| TEXAS INSTRUMENTS INCORPORATED
| Standard Linear and Logic Group
| IBIS Model of SN74CBT16292
| 12-BIT 1-OF-2 FET MULTIPLEXER/DEMULTIPLEXER WITH INTERNAL PULLDOWN RESISTORS
| This file contains package information for the following:
|  TSSOP 56-pin (DGG) package as [Component] CBT16292_DGG
|  TVSOP 56-pin (DGV) package as [Component] CBT16292_DGV
|  SSOP 56-pin (DL) package as [Component] CBT16292_DL
| This device can be powered at the following Vccs:
|  4 volt Vcc
|  5 volt Vcc
| This file provides unique models under the [Model Selector] for each Vcc.
| For operation at a specific Vcc, select the appropriate model after each
| [Model Selector] keyword.
[IBIS Ver]   3.2
[Comment char]  |_char
[File Name]   sn74cbt16292.ibs
[File Rev]   1.1 | b_die
[Date]   January 16, 2004
[Source]   Data created from TI-SPICE simulations at TI-SLL.
[Notes]   The following is an IBIS list for the CBT16292.
   Please contact sllibis@ti.com with questions and
   comments concerning SLL IBIS models.
   - Power-clamp data has been deleted from the input model
   since there is no power-clamp diode.
   - Power Clamp never becomes zero due to internal pulldown
   resistors.
   - Non-monotonic data due to FET characteristics.
[Disclaimer] Property of Texas Instruments Incorporated.  Unauthorized
   reproduction and/or distribution is strictly prohibited.
   This product is protected under copyright law.
   Created  2002, (C) Copyright  2002, Texas Instruments
   Incorporated, All Rights Reserved
   UNLESS THERE IS A SIGNED, WRITTEN AGREEMENT TO THE
   CONTRARY, TEXAS INSTRUMENTS (TI) IS PROVIDING THE IBIS
   MODELS  AND WITHOUT ANY WARRANTY, EXPRESSED OR
   IMPLIED.  TI assumes no liability for:
   1) the accuracy of the IBIS models provided to your
   company;
   2) the proper functioning of these IBIS Models in your
   design or for any resulting applications; or
   3) infringement of patents, copyrights or intellectual
   property rights resulting from your use of these IBIS
   models.
   TI provides IBIS Models as a service to our customers.
   You and your company shall not distribute, sell or give
   these models to anyone else without prior written
   permission from TI.
   TI reserves the right to make changes to our products or
   to discontinue any semiconductor product or service
   without notice, and advises our customers to obtain the
   latest version of relevant information to verify, before
   placing orders, that the information being relied on is
   current.
   Please be aware that your receipt and use of the IBIS
   information provided shall serve as acceptance of these
   terms and conditions.  If you do not accept these terms,
   you should return or destroy the IBIS models and any
   other accompanying information immediately.
| Component CBT16292_DGG 56-pin TSSOP
[Component]   CBT16292_DGG
[Manufacturer]   Texas Instruments, Inc.
[Package]
|   typ   min   max
R_pkg   4.500e-02   3.500e-02   6.200e-02
L_pkg   3.324e-09   2.403e-09   5.094e-09
C_pkg   5.640e-13   3.410e-13   9.140e-13
[Pin]   signal_name   model_name   R_pin   L_pin   C_pin
1   S   CBT16292_IN   6.200e-02   5.094e-09   8.560e-13
2   1A   CBT16292_IO   6.100e-02   4.621e-09   9.020e-13
3   NC   NC   6.000e-02   4.316e-09   8.020e-13
4   2A   CBT16292_IO   5.900e-02   3.968e-09   6.980e-13
5   NC   NC   5.700e-02   3.716e-09   6.490e-13
6   3A   CBT16292_IO   4.200e-02   3.517e-09   6.520e-13
7   NC   NC   4.100e-02   3.160e-09   5.700e-13
8   GND   GND   3.900e-02   2.981e-09   4.820e-13
9   4A   CBT16292_IO   3.900e-02   2.809e-09   4.470e-13
10   NC   NC   3.800e-02   2.715e-09   4.090e-13
11   5A   CBT16292_IO   4.100e-02   2.675e-09   3.910e-13
12   NC   NC   3.900e-02   2.536e-09   3.660e-13
13   6A   CBT16292_IO   3.900e-02   2.457e-09   3.480e-13
14   NC   NC   3.800e-02   2.411e-09   3.530e-13
15   7A   CBT16292_IO   3.900e-02   2.456e-09   3.550e-13
16   NC   NC   3.900e-02   2.471e-09   3.490e-13
17   VCC   POWER   4.000e-02   2.580e-09   3.700e-13
18   8A   CBT16292_IO   3.800e-02   2.651e-09   3.890e-13
19   GND   GND   3.800e-02   2.739e-09   4.110e-13
20   NC   NC   3.900e-02   2.838e-09   4.490e-13
21   9A   CBT16292_IO   3.800e-02   2.988e-09   4.840e-13
22   NC   NC   3.800e-02   3.105e-09   5.640e-13
23   10A   CBT16292_IO   4.000e-02   3.427e-09   6.380e-13
24   NC   NC   5.600e-02   3.654e-09   6.410e-13
25   11A   CBT16292_IO   5.700e-02   3.932e-09   7.000e-13
26   NC   NC   5.800e-02   4.257e-09   8.060e-13
27   12A   CBT16292_IO   5.700e-02   4.580e-09   9.140e-13
28   NC   NC   5.900e-02   5.038e-09   8.610e-13
29   12B2   CBT16292_IO   6.000e-02   5.058e-09   8.580e-13
30   12B1   CBT16292_IO   5.600e-02   4.543e-09   9.040e-13
31   11B2   CBT16292_IO   5.700e-02   4.240e-09   8.030e-13
32   11B1   CBT16292_IO   5.700e-02   3.929e-09   7.000e-13
33   10B2   CBT16292_IO   5.600e-02   3.616e-09   6.370e-13
34   10B1   CBT16292_IO   3.700e-02   3.368e-09   6.400e-13
35   9B2   CBT16292_IO   3.600e-02   3.024e-09   5.630e-13
36   9B1   CBT16292_IO   3.500e-02   2.876e-09   4.740e-13
37   8B2   CBT16292_IO   3.500e-02   2.745e-09   4.440e-13
38   GND   GND   3.700e-02   2.683e-09   4.050e-13
39   8B1   CBT16292_IO   3.800e-02   2.603e-09   3.820e-13
40   7B2   CBT16292_IO   3.800e-02   2.510e-09   3.620e-13
41   7B1   CBT16292_IO   3.600e-02   2.412e-09   3.410e-13
42   6B2   CBT16292_IO   3.800e-02   2.416e-09   3.490e-13
43   6B1   CBT16292_IO   3.700e-02   2.403e-09   3.490e-13
44   5B2   CBT16292_IO   3.700e-02   2.429e-09   3.410e-13
45   5B1   CBT16292_IO   3.600e-02   2.482e-09   3.580e-13
46   4B2   CBT16292_IO   3.700e-02   2.615e-09   3.810e-13
47   4B1   CBT16292_IO   3.500e-02   2.669e-09   4.020e-13
48   3B2   CBT16292_IO   3.600e-02   2.763e-09   4.420e-13
49   GND   GND   3.600e-02   2.942e-09   4.780e-13
50   3B1   CBT16292_IO   3.500e-02   3.053e-09   5.640e-13
51   2B2   CBT16292_IO   3.600e-02   3.409e-09   6.410e-13
52   2B1   CBT16292_IO   5.800e-02   3.698e-09   6.410e-13
53   1B2   CBT16292_IO   5.900e-02   3.975e-09   6.970e-13
54   1B1   CBT16292_IO   6.100e-02   4.327e-09   8.020e-13
55   NC   NC   6.100e-02   4.624e-09   9.050e-13
56   NC   NC   6.000e-02   5.063e-09   8.580e-13
| Component CBT16292_DGV 56-pin TVSOP
[Component]   CBT16292_DGV
[Manufacturer]   Texas Instruments, Inc.
[Package]
|   typ   min   max
R_pkg   6.300e-02   5.000e-02   8.600e-02
L_pkg   2.945e-09   2.392e-09   3.938e-09
C_pkg   3.910e-13   2.710e-13   5.880e-13
[Pin]   signal_name   model_name   R_pin   L_pin   C_pin
1   S   CBT16292_IN   6.800e-02   3.933e-09   5.880e-13
2   1A   CBT16292_IO   6.800e-02   3.569e-09   5.860e-13
3   NC   NC   7.600e-02   3.464e-09   5.150e-13
4   2A   CBT16292_IO   8.600e-02   3.451e-09   4.580e-13
5   NC   NC   8.200e-02   3.278e-09   4.260e-13
6   3A   CBT16292_IO   7.700e-02   3.143e-09   3.870e-13
7   NC   NC   6.900e-02   2.971e-09   4.010e-13
8   GND   GND   5.000e-02   2.787e-09   3.790e-13
9   4A   CBT16292_IO   5.100e-02   2.686e-09   3.200e-13
10   NC   NC   5.200e-02   2.607e-09   3.160e-13
11   5A   CBT16292_IO   5.300e-02   2.497e-09   2.970e-13
12   NC   NC   5.400e-02   2.438e-09   2.920e-13
13   6A   CBT16292_IO   5.500e-02   2.412e-09   2.860e-13
14   NC   NC   5.500e-02   2.400e-09   2.730e-13
15   7A   CBT16292_IO   5.500e-02   2.402e-09   2.730e-13
16   NC   NC   5.400e-02   2.398e-09   2.840e-13
17   VCC   POWER   5.400e-02   2.407e-09   2.890e-13
18   8A   CBT16292_IO   5.300e-02   2.448e-09   2.930e-13
19   GND   GND   5.200e-02   2.548e-09   3.110e-13
20   NC   NC   5.100e-02   2.623e-09   3.160e-13
21   9A   CBT16292_IO   5.000e-02   2.725e-09   3.700e-13
22   NC   NC   6.500e-02   2.903e-09   3.940e-13
23   10A   CBT16292_IO   7.300e-02   3.086e-09   3.870e-13
24   NC   NC   8.200e-02   3.272e-09   4.280e-13
25   11A   CBT16292_IO   8.200e-02   3.394e-09   4.570e-13
26   NC   NC   7.100e-02   3.374e-09   5.080e-13
27   12A   CBT16292_IO   6.900e-02   3.572e-09   5.810e-13
28   NC   NC   6.900e-02   3.937e-09   5.740e-13
29   12B2   CBT16292_IO   6.900e-02   3.923e-09   5.690e-13
30   12B1   CBT16292_IO   6.800e-02   3.546e-09   5.740e-13
31   11B2   CBT16292_IO   7.400e-02   3.422e-09   5.180e-13
32   11B1   CBT16292_IO   8.100e-02   3.395e-09   4.680e-13
33   10B2   CBT16292_IO   8.000e-02   3.255e-09   4.310e-13
34   10B1   CBT16292_IO   7.100e-02   3.063e-09   3.860e-13
35   9B2   CBT16292_IO   6.100e-02   2.878e-09   3.900e-13
36   9B1   CBT16292_IO   5.000e-02   2.709e-09   3.640e-13
37   8B2   CBT16292_IO   5.100e-02   2.607e-09   3.110e-13
38   GND   GND   5.100e-02   2.532e-09   3.060e-13
39   8B1   CBT16292_IO   5.300e-02   2.440e-09   2.890e-13
40   7B2   CBT16292_IO   5.300e-02   2.399e-09   2.860e-13
41   7B1   CBT16292_IO   5.400e-02   2.392e-09   2.820e-13
42   6B2   CBT16292_IO   5.500e-02   2.399e-09   2.710e-13
43   6B1   CBT16292_IO   5.500e-02   2.395e-09   2.710e-13
44   5B2   CBT16292_IO   5.500e-02   2.403e-09   2.830e-13
45   5B1   CBT16292_IO   5.400e-02   2.421e-09   2.880e-13
46   4B2   CBT16292_IO   5.300e-02   2.472e-09   2.920e-13
47   4B1   CBT16292_IO   5.100e-02   2.569e-09   3.090e-13
48   3B2   CBT16292_IO   5.100e-02   2.636e-09   3.130e-13
49   GND   GND   5.000e-02   2.739e-09   3.660e-13
50   3B1   CBT16292_IO   6.500e-02   2.922e-09   3.900e-13
51   2B2   CBT16292_IO   7.200e-02   3.076e-09   3.840e-13
52   2B1   CBT16292_IO   8.100e-02   3.249e-09   4.300e-13
53   1B2   CBT16292_IO   8.300e-02   3.400e-09   4.550e-13
54   1B1   CBT16292_IO   7.300e-02   3.421e-09   5.060e-13
55   NC   NC   6.900e-02   3.579e-09   5.780e-13
56   NC   NC   6.900e-02   3.938e-09   5.810e-13
| Component CBT16292_DL 56-pin SSOP
[Component]   CBT16292_DL
[Manufacturer]   Texas Instruments, Inc.
[Package]
|   typ   min   max
R_pkg   5.500e-02   4.800e-02   6.700e-02
L_pkg   6.539e-09   4.802e-09   9.746e-09
C_pkg   1.880e-13   7.600e-14   5.170e-13
[Pin]   signal_name   model_name   R_pin   L_pin   C_pin
1   S   CBT16292_IN   6.400e-02   9.646e-09   5.130e-13
2   1A   CBT16292_IO   5.900e-02   8.723e-09   2.700e-13
3   NC   NC   5.900e-02   8.139e-09   2.230e-13
4   2A   CBT16292_IO   5.600e-02   7.554e-09   2.010e-13
5   NC   NC   5.400e-02   6.991e-09   1.950e-13
6   3A   CBT16292_IO   5.300e-02   6.659e-09   2.020e-13
7   NC   NC   5.500e-02   6.321e-09   2.070e-13
8   GND   GND   5.500e-02   5.942e-09   1.330e-13
9   4A   CBT16292_IO   5.700e-02   5.767e-09   1.320e-13
10   NC   NC   5.400e-02   5.459e-09   1.210e-13
11   5A   CBT16292_IO   5.100e-02   5.224e-09   1.400e-13
12   NC   NC   4.800e-02   5.088e-09   1.260e-13
13   6A   CBT16292_IO   5.000e-02   5.021e-09   9.600e-14
14   NC   NC   5.100e-02   4.802e-09   7.600e-14
15   7A   CBT16292_IO   5.100e-02   4.803e-09   7.600e-14
16   NC   NC   5.000e-02   5.021e-09   9.600e-14
17   VCC   POWER   4.800e-02   5.088e-09   1.260e-13
18   8A   CBT16292_IO   5.100e-02   5.224e-09   1.400e-13
19   GND   GND   5.400e-02   5.459e-09   1.210e-13
20   NC   NC   5.700e-02   5.768e-09   1.330e-13
21   9A   CBT16292_IO   5.500e-02   5.942e-09   1.330e-13
22   NC   NC   5.500e-02   6.320e-09   2.060e-13
23   10A   CBT16292_IO   5.300e-02   6.659e-09   2.030e-13
24   NC   NC   5.400e-02   6.991e-09   1.960e-13
25   11A   CBT16292_IO   5.600e-02   7.554e-09   2.010e-13
26   NC   NC   5.900e-02   8.139e-09   2.230e-13
27   12A   CBT16292_IO   5.900e-02   8.727e-09   2.700e-13
28   NC   NC   6.700e-02   9.746e-09   5.170e-13
29   12B2   CBT16292_IO   6.300e-02   9.630e-09   5.110e-13
30   12B1   CBT16292_IO   6.000e-02   8.751e-09   2.710e-13
31   11B2   CBT16292_IO   6.000e-02   8.184e-09   2.250e-13
32   11B1   CBT16292_IO   5.600e-02   7.543e-09   2.000e-13
33   10B2   CBT16292_IO   5.400e-02   7.005e-09   1.960e-13
34   10B1   CBT16292_IO   5.600e-02   6.714e-09   2.040e-13
35   9B2   CBT16292_IO   5.800e-02   6.384e-09   2.080e-13
36   9B1   CBT16292_IO   5.700e-02   5.976e-09   1.340e-13
37   8B2   CBT16292_IO   5.700e-02   5.743e-09   1.300e-13
38   GND   GND   5.400e-02   5.468e-09   1.190e-13
39   8B1   CBT16292_IO   5.500e-02   5.328e-09   1.420e-13
40   7B2   CBT16292_IO   5.200e-02   5.189e-09   1.290e-13
41   7B1   CBT16292_IO   5.200e-02   5.053e-09   9.600e-14
42   6B2   CBT16292_IO   5.100e-02   4.825e-09   7.600e-14
43   6B1   CBT16292_IO   5.400e-02   4.896e-09   7.800e-14
44   5B2   CBT16292_IO   5.200e-02   5.093e-09   9.700e-14
45   5B1   CBT16292_IO   5.100e-02   5.179e-09   1.280e-13
46   4B2   CBT16292_IO   5.400e-02   5.314e-09   1.420e-13
47   4B1   CBT16292_IO   5.500e-02   5.511e-09   1.210e-13
48   3B2   CBT16292_IO   5.700e-02   5.771e-09   1.310e-13
49   GND   GND   5.600e-02   5.957e-09   1.330e-13
50   3B1   CBT16292_IO   5.500e-02   6.320e-09   2.060e-13
51   2B2   CBT16292_IO   5.200e-02   6.621e-09   2.000e-13
52   2B1   CBT16292_IO   5.300e-02   6.973e-09   1.950e-13
53   1B2   CBT16292_IO   5.700e-02   7.571e-09   2.020e-13
54   1B1   CBT16292_IO   5.700e-02   8.097e-09   2.220e-13
55   NC   NC   5.900e-02   8.723e-09   2.710e-13
56   NC   NC   6.100e-02   9.560e-09   5.090e-13
[Series Switch Groups]
| Function Group States
On  1 /   | 1A->1B1 S LOW
On  2 /   | 1A->1B2 S HIGH
[Series Pin Mapping]   pin_2   model_name   function_table_group
2   54   CBT16292_IO_40_S   1
| 2   54   CBT16292_IO_50_S   1
2   53   CBT16292_IO_40_S   2
| 2   53   CBT16292_IO_50_S   2
4   52   CBT16292_IO_40_S   1
| 4   52   CBT16292_IO_50_S   1
4   51   CBT16292_IO_40_S   2
| 4   51   CBT16292_IO_50_S   2
6   50   CBT16292_IO_40_S   1
| 6   50   CBT16292_IO_50_S   1
6   48   CBT16292_IO_40_S   2
| 6   48   CBT16292_IO_50_S   2
9   47   CBT16292_IO_40_S   1
| 9   47   CBT16292_IO_50_S   1
9   46   CBT16292_IO_40_S   2
| 9   46   CBT16292_IO_50_S   2
11   45   CBT16292_IO_40_S   1
| 11   45   CBT16292_IO_50_S   1
11   44   CBT16292_IO_40_S   2
| 11   44   CBT16292_IO_50_S   2
13   43   CBT16292_IO_40_S   1
| 13   43   CBT16292_IO_50_S   1
13   42   CBT16292_IO_40_S   2
| 13   42   CBT16292_IO_50_S   2
15   41   CBT16292_IO_40_S   1
| 15   41   CBT16292_IO_50_S   1
15   40   CBT16292_IO_40_S   2
| 15   40   CBT16292_IO_50_S   2
18   39   CBT16292_IO_40_S   1
| 18   39   CBT16292_IO_50_S   1
18   37   CBT16292_IO_40_S   2
| 18   37   CBT16292_IO_50_S   2
21   36   CBT16292_IO_40_S   1
| 21   36   CBT16292_IO_50_S   1
21   35   CBT16292_IO_40_S   2
| 21   35   CBT16292_IO_50_S   2
23   34   CBT16292_IO_40_S   1
| 23   34   CBT16292_IO_50_S   1
23   33   CBT16292_IO_40_S   2
| 23   33   CBT16292_IO_50_S   2
25   32   CBT16292_IO_40_S   1
| 25   32   CBT16292_IO_50_S   1
25   31   CBT16292_IO_40_S   2
| 25   31   CBT16292_IO_50_S   2
27   30   CBT16292_IO_40_S   1
| 27   30   CBT16292_IO_50_S   1
27   29   CBT16292_IO_40_S   2
| 27   29   CBT16292_IO_50_S   2
| Model CBT16292_IN
[Model Selector]   CBT16292_IN
CBT16292_IN_40   4 volt Vcc
CBT16292_IN_50   5 volt Vcc
| Model CBT16292_IO
[Model Selector]   CBT16292_IO
CBT16292_IO_40   4 volt Vcc
CBT16292_IO_50   5 volt Vcc
| Model CBT16292_IO_S
[Model Selector]   CBT16292_IO_S
CBT16292_IO_40_S   4 volt Vcc
CBT16292_IO_50_S   5 volt Vcc
[Model]   CBT16292_IO_40_S
Model_type  Series_switch
| variable   typ   min   max
C_comp   0   0   0
[Temperature Range]   40   100   -40
| Ambient temperature   25   85   -40
[Voltage range]   4   4   4
[On]
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[Off]
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[Model]   CBT16292_IO_50_S
Model_type  Series_switch
| variable   typ   min   max
C_comp   0   0   0
[Temperature Range]   40   100   -40
| Ambient temperature   25   85   -40
[Voltage range]   5   4.5   5.5
[On]
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[Off]
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| Models and submodels in the file (6): CBT16292_IN_40 (Input), CBT16292_IN_50 (Input), CBT16292_IO_40_S (Series_switch), CBT16292_IO_40 (Terminator), CBT16292_IO_50_S (Series_switch), CBT16292_IO_50 (Terminator)
